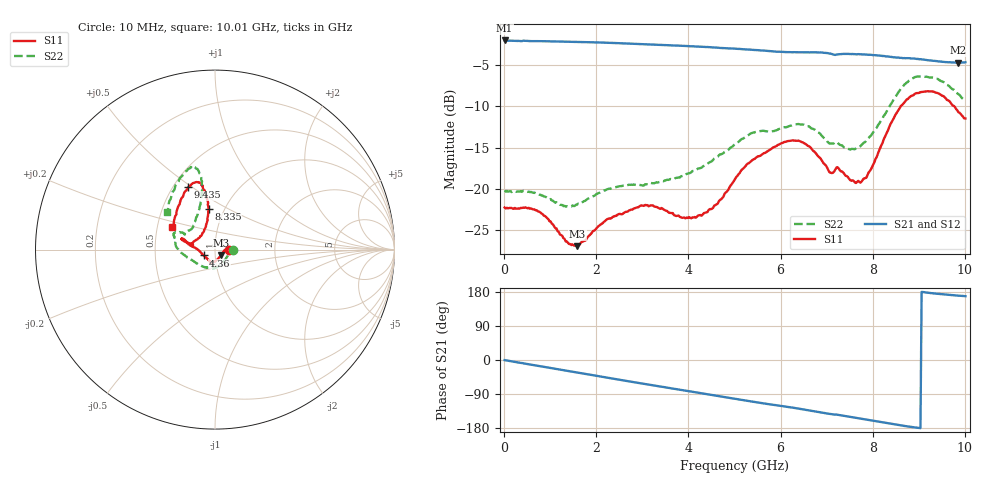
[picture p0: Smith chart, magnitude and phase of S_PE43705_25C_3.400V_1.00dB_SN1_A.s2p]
! Device ID: PE43705
! Serial: 1
! Insertion: A
! Impedance: 50 ohm
! Temp: 25C
! VDD: 3.400V
! Attenuation Step: 1.00dB
#  Hz  S  RI  R  50
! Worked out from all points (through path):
!   401 points, 10 MHz to 10.01 GHz, reference 50 ohm
!   highest |S21| = -2.00 dB at 10 MHz (marker M1); lowest = -4.7 dB at 9.86 GHz (marker M2)
!   group delay of S21, straight-line fit = 54.4 ps
!   lowest |S11| = -27.0 dB at 1.585 GHz (marker M3), VSWR 1.09, Z = 53.4 - j3.22 ohm
!   |S11| at or under -10 dB: start of sweep to 8.603 GHz; 9.77 GHz to end of sweep
!   |S22| runs from -22.2 to -6.4 dB; largest |S21 - S12| = 0.0067
!   S11 on the Smith chart (normalised r, x): 10 MHz: 1.17, -0.00; 4.36 GHz: 0.88, -0.06; 8.335 GHz: 0.84, +0.40; 9.435 GHz: 0.59, +0.48; 10.01 GHz: 0.60, +0.16
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1e7  0.0771 -0.000513  0.7944 -0.00406  0.7946 -0.0035  0.0978 -0.000648
7.35e8  0.0708 0.0175  0.758 -0.2093  0.7582 -0.209  0.0925 0.00488
1.585e9  0.0334 -0.0301  0.6522 -0.4256  0.6524 -0.4258  0.0553 -0.0582
1.685e9  0.0285 -0.0385  0.6358 -0.4484  0.6358 -0.4486  0.0476 -0.0675
2.26e9  0.000845 -0.0658  0.5232 -0.5634  0.5235 -0.563  0.00735 -0.0996
3.01e9  -0.0206 -0.0763  0.3477 -0.6679  0.3487 -0.6672  -0.0338 -0.0992
3.36e9  -0.0247 -0.0724  0.2628 -0.6986  0.2636 -0.6978  -0.0458 -0.0999
3.885e9  -0.0385 -0.0547  0.1284 -0.7252  0.129 -0.7246  -0.0806 -0.0889
4.36e9  -0.0638 -0.0325  0.00587 -0.7252  0.00657 -0.7257  -0.1247 -0.0614
5.01e9  -0.1141 0.0117  -0.1523 -0.6912  -0.1517 -0.6912  -0.1856 -0.0189
6.06e9  -0.1811 0.0614  -0.3592 -0.5733  -0.3575 -0.5733  -0.2258 0.0682
6.685e9  -0.1672 0.0439  -0.4684 -0.4832  -0.4687 -0.4827  -0.2106 0.0973
7.085e9  -0.1226 0.0258  -0.5251 -0.4016  -0.5257 -0.4025  -0.1688 0.0845
7.26e9  -0.1282 0.0352  -0.5361 -0.3767  -0.5343 -0.3778  -0.1585 0.1001
7.685e9  -0.0828 0.0751  -0.5881 -0.2919  -0.5873 -0.2922  -0.121 0.1328
7.91e9  -0.0599 0.1105  -0.6042 -0.2404  -0.6047 -0.2441  -0.1063 0.1739
8.335e9  -0.0359 0.2253  -0.6173 -0.144  -0.6152 -0.1482  -0.0735 0.2974
8.36e9  -0.037 0.2357  -0.6179 -0.1385  -0.616 -0.1415  -0.0744 0.3075
8.86e9  -0.0772 0.3605  -0.6164 -0.0317  -0.6129 -0.0339  -0.1078 0.4539
9.435e9  -0.1488 0.348  -0.5897 0.0589  -0.5879 0.0589  -0.1749 0.4235
9.86e9  -0.2146 0.1969  -0.5732 0.1036  -0.5733 0.1023  -0.2479 0.2814
1.001e10  -0.2373 0.1233  -0.5743 0.1176  -0.5768 0.1144  -0.2688 0.2116
